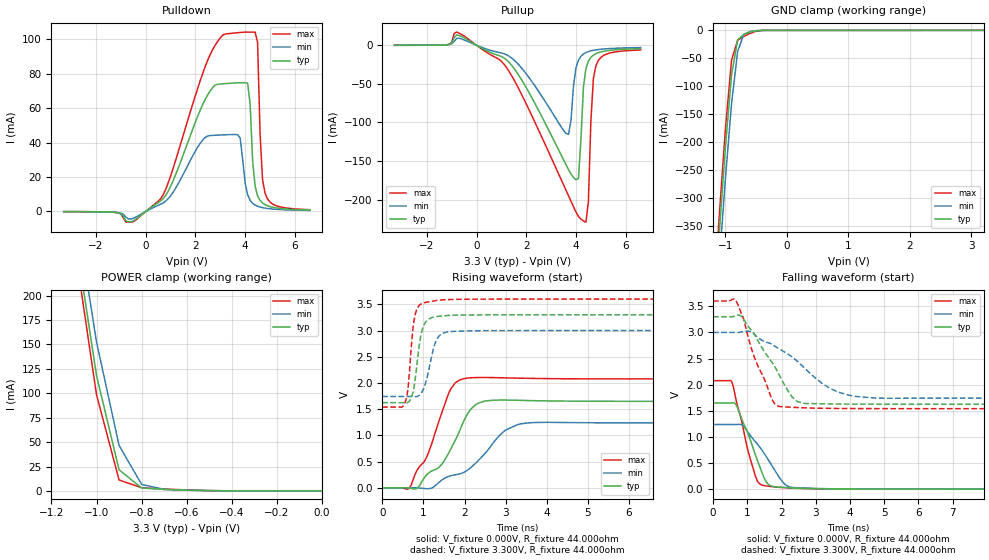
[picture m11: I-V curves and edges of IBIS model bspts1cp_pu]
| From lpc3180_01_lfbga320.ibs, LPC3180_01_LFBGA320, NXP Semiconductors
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| |   Rev 0.20 IBIS Model Design Automation Generation   |
| |   N O N - S I L I C O N   C O R R E L A T E D   |
| |   This IBIS [Model] is pre-Beta tactical support   |
| |  Note: this IBIS [Model] contains clamp curves generated   |
| |   through simulation which should not be relied upon   |
| bspts1cp
|   Bidirectional Pad 3v3
|   3state Output
|   Plain Input
|   1ns Slew Rate control
|   CMOS
|   Programmable between
|   - (p1=0, p2=1) plain input
|   - (p1=0, p2=0) with Pull Up
|   - (p1=1, p2=1) with Pull Down
|   - (p1=1, p2=0) with Repeater
|   Characterized at Core 1.2V and I/O 3.3V
| Pull Up Mode (p1=0, p2=0)
[Model]   bspts1cp_pu | of bspts1cp
Model_type   I/O
Polarity   Non-Inverting
Enable   Active-Low
|  Reciever Thresholds
Vinl   = 0.36V
Vinh   = 0.84V
| AC Test Load Conditions
Vref   = 0
Cref   = 1.2e-11
Rref   = 1000000000
Vmeas   = 0.6
| [Process Range]   typical   min   max
| C_comp edge width   400.000ps   400.000ps   400.000ps
| C_comp Tstrobe   40.000fs   40.000fs   40.000fs
C_comp   2.381pF   2.241pF   2.551pF
[Temperature Range]   25   125   -40
[Voltage Range]   3.30V   3.00V   3.60V
[GND Clamp Reference]   0.00V   0.00V   0.00V
[Pulldown Reference]   0.00V   0.00V   0.00V
[POWER Clamp Reference]   3.30V   3.00V   3.60V
[Pullup Reference]   3.30V   3.00V   3.60V
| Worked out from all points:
|   slope of the pulldown table from 0 to 0.495 V, typ, clamps not added: 97.1 ohm
|   slope of the pullup table from 0 to 0.495 V, typ, clamps not added: 59.3 ohm
|   GND clamp passes 1 mA (typ) near -0.51 V on its own axis
|   POWER clamp passes 1 mA (typ) near -0.63 V on its own axis
|   rising waveform, V_fixture 0.000V, R_fixture 44.000ohm: 20-80 % time 782ps typ, 1.07ns min, 630ps max; typ from 0.001 V to 1.65 V
|   falling waveform, V_fixture 0.000V, R_fixture 44.000ohm: 20-80 % time 570ps typ, 781ps min, 473ps max; typ from 1.65 V to 0.001 V
|   rising waveform, V_fixture 3.300V, R_fixture 44.000ohm: 20-80 % time 175ps typ, 230ps min, 140ps max; typ from 1.62 V to 3.3 V
|   falling waveform, V_fixture 3.300V, R_fixture 44.000ohm: 20-80 % time 910ps typ, 1.48ns min, 670ps max; typ from 3.3 V to 1.62 V
[GND Clamp]
| ref voltage   0.00V   0.00V   0.00V
|   Voltage   I(typ)   I(min)   I(max)
-3.3V     -4.198A    -4.223A    -4.188A
-1.2V     -526mA     -577.5mA   -497.2mA
-1.1V     -363.6mA   -417.9mA   -332.6mA
-1V       -210.1mA   -266.3mA   -177.3mA
-900mV    -79.72mA   -131.5mA   -53.31mA
-800mV    -16.78mA   -37.39mA   -17.84mA
-700mV    -7.182mA   -7.273mA   -10.95mA
-600mV    -3.024mA   -2.214mA   -5.482mA
-500mV    -725.7uA   -585.9uA   -1.656mA
-400mV    -110.5uA   -112.8uA   -213.4uA
3.2V      -4.082uA   6.375uA    -21.05uA
[Power Clamp]   | Vtable = Vcc - Vpad
| ref voltage   3.30V   3.00V   3.60V
|   Voltage   I(typ)   I(min)   I(max)
-3.3V     4.52A      4.504A     4.537A
-1.1V     269.9mA    299.6mA    255.3mA
-1V       118.1mA    152.4mA    98.46mA
-900mV    21.6mA     46.51mA    11.21mA
-800mV    3.019mA    6.665mA    3.25mA
-700mV    1.526mA    1.552mA    1.973mA
-600mV    767.7uA    705uA      1.011mA
-400mV    58.36uA    81.92uA    64.04uA
0V        755.1pA    5.591nA    627.9pA
[Pulldown]
| ref voltage   0.00V   0.00V   0.00V
|   Voltage   I(typ)   I(min)   I(max)
-3.3V     -80.68uA   -69.9uA    -74.32uA
-600mV    -5.92mA    -4.329mA   -6.173mA
500mV     5.147mA    3.568mA    5.923mA
2.5V      67.8mA     43.83mA    87.99mA
3.7V      74.65mA    44.53mA    103.7mA
4V        74.69mA    16.44mA    104.1mA
4.2V      62.38mA    6.514mA    104mA
4.3V      29.48mA    4.769mA    104mA
4.5V      9.068mA    3.068mA    98.17mA
4.6V      6.413mA    2.587mA    45.14mA
4.8V      3.956mA    1.96mA     10.6mA
6.6V      844.8uA    597.5uA    1.056mA
[Pullup]   | Vtable = Vcc - Vpad
| ref voltage   3.30V   3.00V   3.60V
|   Voltage   I(typ)   I(min)   I(max)
-3.3V     39.4uA     37.84uA    38.83uA
-800mV    13.66mA    9.123mA    17.15mA
1V        -14.52mA   -9.936mA   -20.86mA
3.7V      -161.3mA   -115.5mA   -195.1mA
4V        -174.4mA   -29.02mA   -216.2mA
4.1V      -172.4mA   -19.17mA   -221.9mA
4.4V      -30.01mA   -9.422mA   -229.4mA
4.5V      -20.4mA    -8.135mA   -202.5mA
4.6V      -15.61mA   -7.195mA   -97.93mA
4.7V      -12.75mA   -6.481mA   -42.99mA
4.8V      -10.87mA   -5.92mA    -26.67mA
6.6V      -4.278mA   -2.929mA   -6.056mA
[Ramp]
R_load   = 44.000ohm
|   dV/dt(typ)   dV/dt(min)   dV/dt(max)
dV/dt_r   1.003V/795.000ps   754.410mV/1.105ns   1.260V/635.000ps
dV/dt_f   1.021V/900.000ps   769.092mV/1.445ns   1.253V/655.000ps
[Rising Waveform]  | cubic spline decimation from 2001 points
V_fixture   = 0.000V
R_fixture   = 44.000ohm
|   Time   V(typ)   V(min)   V(max)
0s        1.464mV    895.4uV    2.142mV
655ps     -3.065mV   1.321mV    -6.652mV
1.09ns    257.7mV    -16.32mV   605.8mV
1.44ns    444.1mV    144.6mV    1.416V
1.67ns    745.8mV    232mV      1.892V
1.96ns    1.234V     287.7mV    2.076V
2.43ns    1.642V     598.6mV    2.105V
2.935ns   1.674V     1.062V     2.099V
3.45ns    1.667V     1.23V      2.09V
10ns      1.65V      1.238V     2.077V
[Falling Waveform]  | cubic spline decimation from 2001 points
V_fixture   = 0.000V
R_fixture   = 44.000ohm
|   Time   V(typ)   V(min)   V(max)
0s        1.65V      1.238V     2.077V
550ps     1.651V     1.238V     2.047V
710ps     1.567V     1.239V     1.602V
1.2ns     726.4mV    936.9mV    331.8mV
1.31ns    527.5mV    851.4mV    141.8mV
1.45ns    285.6mV    726.7mV    75.56mV
1.69ns    63.98mV    481.8mV    51.38mV
2.075ns   33.74mV    109.2mV    29.64mV
2.34ns    23.56mV    32.76mV    20.59mV
10ns      1.465mV    896.3uV    2.143mV
[Rising Waveform]  | cubic spline decimation from 2001 points
V_fixture   = 3.300V
V_fixture_min = 3.000V
V_fixture_max = 3.600V
R_fixture   = 44.000ohm
|   Time   V(typ)   V(min)   V(max)
0s        1.625V     1.743V     1.541V
555ps     1.623V     1.743V     1.631V
625ps     1.631V     1.743V     1.892V
730ps     1.77V      1.742V     2.906V
785ps     1.982V     1.74V      3.244V
920ps     2.824V     1.778V     3.494V
1.005ns   3.092V     1.89V      3.527V
1.31ns    3.265V     2.805V     3.572V
1.58ns    3.286V     2.972V     3.589V
10ns      3.3V       3V         3.6V
[Falling Waveform]  | cubic spline decimation from 2001 points
V_fixture   = 3.300V
V_fixture_min = 3.000V
V_fixture_max = 3.600V
R_fixture   = 44.000ohm
|   Time   V(typ)   V(min)   V(max)
0s        3.3V       3V         3.6V
670ps     3.322V     2.999V     3.604V
840ps     3.3V       3.01V      3.346V
1.255ns   2.908V     2.935V     2.444V
1.725ns   2.425V     2.771V     1.718V
1.9ns     2.23V      2.698V     1.589V
2.47ns    1.675V     2.444V     1.562V
3.4ns     1.632V     1.936V     1.547V
4.135ns   1.627V     1.777V     1.543V
10ns      1.625V     1.743V     1.541V
